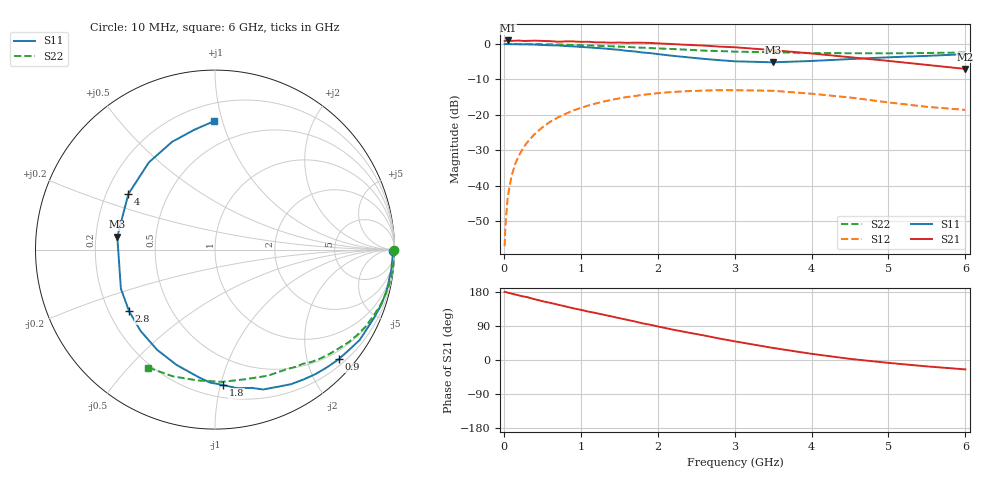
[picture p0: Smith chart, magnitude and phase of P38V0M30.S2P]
! SIEMENS Small Signal Semiconductors
! BFP181
! Si NPN RF Bipolar Junction Transistor in SOT143
! VCE = 8 V  IC = 0.3 mA
! Common Emitter S-Parameters:  March  1996
# GHz  S  MA  R  50
!  f  S11  S21  S12  S22
! GHz  MAG  ANG  MAG  ANG  MAG  ANG  MAG  ANG
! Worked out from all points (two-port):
!   36 points, 10 MHz to 6 GHz, reference 50 ohm
!   highest |S21| = 0.96 dB at 50 MHz (marker M1); lowest = -7.1 dB at 6 GHz (marker M2)
!   |S21| within 3 dB of the highest: start of sweep to 3.64 GHz
!   lowest |S11| = -5.2 dB at 3.5 GHz (marker M3), VSWR 3.43, Z = 14.6 + j3 ohm
!   |S11| at or under -10 dB: nowhere
!   |S22| runs from -2.7 to 0.0 dB; largest |S21 - S12| = 1.1
!   S11 on the Smith chart (normalised r, x): 10 MHz: open; 900 MHz: 0.32, -2.60; 1.8 GHz: 0.29, -1.02; 2.8 GHz: 0.28, -0.30; 4 GHz: 0.29, +0.27; 6 GHz: 0.32, +0.94
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0.01  0.99 -0.6  1.099 179.8  0.0014 79.7  0.9985 -0.2
0.02  0.9974 -1.0  1.104 179.6  0.0026 83.7  0.9983 -0.4
0.05  0.9905 -2.0  1.117 177.7  0.0069 88.8  0.998 -1.2
0.1  0.9888 -4.7  1.103 175.1  0.0137 86.3  0.9977 -2.4
0.15  0.989 -6.9  1.107 172.9  0.0206 84.1  0.9971 -3.5
0.3  0.9824 -13.8  1.1 166.1  0.0403 79.5  0.9952 -7.0
0.4  0.9763 -18.3  1.112 160.3  0.0534 76.5  0.993 -9.3
0.6  0.9548 -27.6  1.092 150.9  0.0794 69.2  0.9841 -13.9
0.9  0.9207 -41.6  1.082 136.6  0.1146 59.0  0.9646 -20.5
1.1  0.8917 -51.0  1.071 127.7  0.1352 52.4  0.9492 -24.8
1.5  0.8243 -71.0  1.046 110.5  0.1702 40.0  0.9138 -32.9
1.8  0.7559 -86.6  1.038 96.9  0.1902 31.5  0.8829 -38.5
2.2  0.6772 -108.5  0.992 80.0  0.2099 20.1  0.845 -45.8
2.6  0.6143 -132.4  0.946 64.9  0.2192 10.0  0.803 -52.4
2.8  0.5888 -144.5  0.915 56.7  0.2221 4.9  0.7921 -55.7
3  0.5676 -157.5  0.896 49.3  0.2218 -0.2  0.7766 -59.1
3.5  0.549 172.5  0.815 31.8  0.2179 -11.1  0.7619 -67.2
4  0.5736 147.3  0.732 16.3  0.1981 -20.3  0.7421 -76.6
4.5  0.6097 127.2  0.648 3.0  0.1751 -27.4  0.7379 -86.9
5  0.6464 111.7  0.575 -7.6  0.1493 -31.0  0.7353 -97.5
5.5  0.6771 99.9  0.505 -16.9  0.1294 -29.4  0.7442 -108.3
6  0.7152 90.5  0.443 -24.8  0.117 -24.8  0.7549 -119.4
